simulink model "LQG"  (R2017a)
settings: Solver=VariableStepAuto  StartTime=0.0  StopTime=10.0  RelTol=1e-3
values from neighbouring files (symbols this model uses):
  baud = 250000    [init.m]    (also in steadyState.m; MISOcontrol.m; MISO_demo.m; runSteptest.m)
  com = 'COM4'    [init.m]    (also in steadyState.m; MISOcontrol.m; MISO_demo.m; runSteptest.m)
  fixed_u1 = 0    [init.m]    (also in MISOcontrol.m; MISO_demo.m; SISOcontrol.m)
  fixed_u2 = 0    [init.m]    (also in MISOcontrol.m; MISO_demo.m; SISOcontrol.m)
  fixed_u3 = 0    [init.m]    (also in MISOcontrol.m; MISO_demo.m; SISOcontrol.m)
  fTf = 0.1    [init.m]    (also in steadyState.m; MISOcontrol.m; MISO_demo.m; runSteptest.m)
  fTl = 0.05    [init.m]    (also in steadyState.m; MISOcontrol.m; MISO_demo.m; runSteptest.m)
  fTt = 0.05    [init.m]    (also in steadyState.m; MISOcontrol.m; MISO_demo.m; runSteptest.m)
  Ts = 0.1    [init.m]    (also in steadyState.m; identification.m; MISOcontrol.m; MISO_demo.m)
  u0 = stst.u    [LightPlantLQG.m]
  x0 = L*stst.y    [LightPlantLQG.m]
undefined symbols (not defined in the file or in its folder): A, B, C, D, K_lqr, L
libraries: tom_lib x1

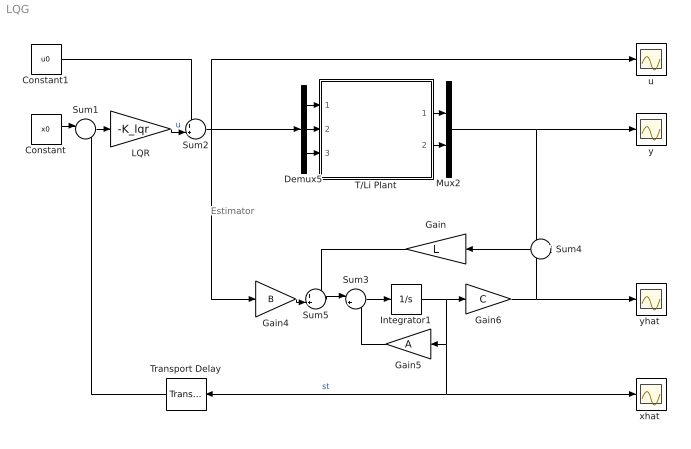
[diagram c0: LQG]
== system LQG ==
  note: Estimator
  Constant : Constant  Value=x0
  Constant1 : Constant  Value=u0
  Demux5 : Demux  Outputs=3
  Gain : Gain  Gain=L  Multiplication=Matrix(K*u)
  Gain4 : Gain  Gain=B  Multiplication=Matrix(K*u)
  Gain5 : Gain  Gain=A  Multiplication=Matrix(K*u)
  Gain6 : Gain  Gain=C  Multiplication=Matrix(K*u)
  Integrator1 : Integrator
  LQR : Gain  Gain=-K_lqr  Multiplication=Matrix(K*u)
  Mux2 : Mux  Inputs=2
  Sum1 : Sum  Inputs=|-+
  Sum2 : Sum  Inputs=++|
  Sum3 : Sum  Inputs=|++
  Sum4 : Sum  Inputs=+-
  Sum5 : Sum  Inputs=++|
  T/Li Plant : Subsystem
  Transport Delay : TransportDelay  DelayTime=0.1
  u : Scope
  "xhat " : Scope
  y : Scope
  "yhat " : Scope
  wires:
  LQR/1 -> Sum2/2  "u"
  Sum1/1 -> LQR/1
  Integrator1/1 -> Gain6/1, Transport Delay/1, "xhat "/1, Gain5/1  "st"
  Gain5/1 -> Sum3/2
  Sum3/1 -> Integrator1/1
  Gain6/1 -> "yhat "/1, Sum4/2
  Gain4/1 -> Sum5/2
  Sum5/1 -> Sum3/1
  Sum4/1 -> Gain/1
  Gain/1 -> Sum5/1
  T/Li Plant/2(LI) -> Mux2/2
  T/Li Plant/1(T) -> Mux2/1
  Demux5/1 -> T/Li Plant/1(B)
  Demux5/3 -> T/Li Plant/3(LED)
  Demux5/2 -> T/Li Plant/2(F)
  Constant/1 -> Sum1/1
  Sum2/1 -> Gain4/1, Demux5/1, u/1
  Constant1/1 -> Sum2/1
  Transport Delay/1 -> Sum1/2
  Mux2/1 -> y/1, Sum4/1

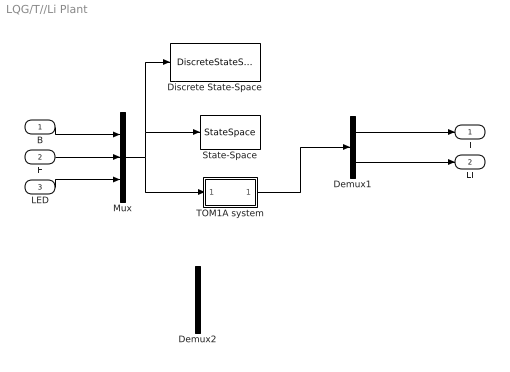
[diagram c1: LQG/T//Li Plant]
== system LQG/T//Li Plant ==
  B : Inport
  F : Inport  Port=2
  LED : Inport  Port=3
  Demux1 : Demux  Outputs=2
  Demux2 : Demux  Commented=on  Outputs=2
  Discrete State-Space : DiscreteStateSpace  Commented=on  A=A  B=B  C=C  D=D  X0=x0  SampleTime=Ts
  Mux : Mux  Inputs=3
  State-Space : StateSpace  Commented=on  A=A  B=B  C=C  D=D  X0=x0
  TOM1A system : Subsystem
  T : Outport
  LI : Outport  Port=2
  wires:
  B/1 -> Mux/1
  F/1 -> Mux/2
  LED/1 -> Mux/3
  Mux/1 -> Discrete State-Space/1, State-Space/1, TOM1A system/1(u)
  ? -> Demux2/1
  Demux1/2 -> LI/1
  Demux1/1 -> T/1
  TOM1A system/1(y) -> Demux1/1

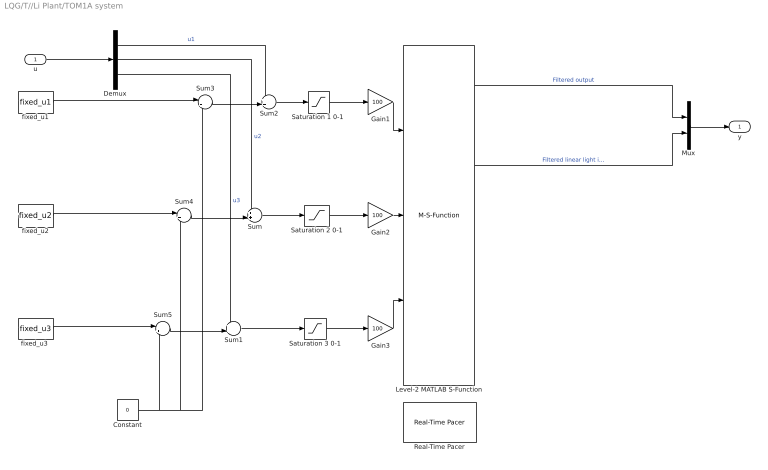
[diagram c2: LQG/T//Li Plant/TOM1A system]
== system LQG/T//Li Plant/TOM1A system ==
  u : Inport
  Constant : Constant  Value=0
  Demux : Demux  Outputs=3
  Gain1 : Gain  Gain=100
  Gain2 : Gain  Gain=100
  Gain3 : Gain  Gain=100
  Level-2 MATLAB S-Function : M-S-Function  FunctionName=tom1ar8  Parameters=Ts,com,baud,fTt,fTl,fTf
  Mux : Mux  Inputs=2
  Real-Time Pacer : tom_lib/Real-Time Pacer  simTimePerRealTime=1
  "Saturation 1 0-1 " : Saturate  UpperLimit=1  LowerLimit=0  ZeroCross=off
  Saturation 2 0-1 : Saturate  UpperLimit=1  LowerLimit=0  ZeroCross=off
  Saturation 3 0-1 : Saturate  UpperLimit=1  LowerLimit=0  ZeroCross=off
  Sum : Sum  Inputs=++|
  Sum1 : Sum  Inputs=++|
  Sum2 : Sum  Inputs=++|
  Sum3 : Sum  Inputs=|++
  Sum4 : Sum  Inputs=|++
  Sum5 : Sum  Inputs=|++
  fixed_u1 : Constant  Value=fixed_u1  SampleTime=Ts
  fixed_u2 : Constant  Value=fixed_u2  SampleTime=Ts
  "fixed_u3 " : Constant  Value=fixed_u3  SampleTime=Ts
  y : Outport
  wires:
  Level-2 MATLAB S-Function/14 -> ?  "Fan filtered  rpm"
  Level-2 MATLAB S-Function/3 -> ?  "Derivative of internal temperature"
  Level-2 MATLAB S-Function/4 -> ?  "Filtered external temperature"
  Level-2 MATLAB S-Function/13 -> ?  "Fan voltage"
  Level-2 MATLAB S-Function/11 -> ?  "Bulb voltage"
  Level-2 MATLAB S-Function/8 -> ?  "Filtered logaritmic light intensity"
  Level-2 MATLAB S-Function/1 -> ?  "Board temperature"
  Level-2 MATLAB S-Function/5 -> ?  "Derivate of external temperature"
  Level-2 MATLAB S-Function/12 -> ?  "Fan current"
  Level-2 MATLAB S-Function/9 -> ?  "Derivate of logaritmic light intensity"
  Level-2 MATLAB S-Function/16 -> ?  "Count of fan rpm"
  Level-2 MATLAB S-Function/15 -> ?  "Derivate of fan rpm"
  Level-2 MATLAB S-Function/10 -> ?  "Bulb current"
  Level-2 MATLAB S-Function/6 -> Mux/2  "Filtered linear light intensity"
  Level-2 MATLAB S-Function/7 -> ?  "Derivate of linear light intensity"
  Demux/1 -> Sum2/1  "u1"
  Demux/2 -> Sum/1  "u2"
  Demux/3 -> Sum1/1  "u3"
  u/1 -> Demux/1
  Level-2 MATLAB S-Function/2 -> Mux/1  "Filtered output"
  Mux/1 -> y/1
  fixed_u1/1 -> Sum3/1
  Sum3/1 -> Sum2/2
  Constant/1 -> Sum5/2, Sum4/2, Sum3/2
  fixed_u2/1 -> Sum4/1
  "fixed_u3 "/1 -> Sum5/1
  Sum5/1 -> Sum1/2
  Sum4/1 -> Sum/2
  Gain1/1 -> Level-2 MATLAB S-Function/1
  Gain2/1 -> Level-2 MATLAB S-Function/2
  Gain3/1 -> Level-2 MATLAB S-Function/3
  Saturation 2 0-1/1 -> Gain2/1
  Sum/1 -> Saturation 2 0-1/1
  Sum2/1 -> "Saturation 1 0-1 "/1
  Saturation 3 0-1/1 -> Gain3/1
  Sum1/1 -> Saturation 3 0-1/1
  "Saturation 1 0-1 "/1 -> Gain1/1
